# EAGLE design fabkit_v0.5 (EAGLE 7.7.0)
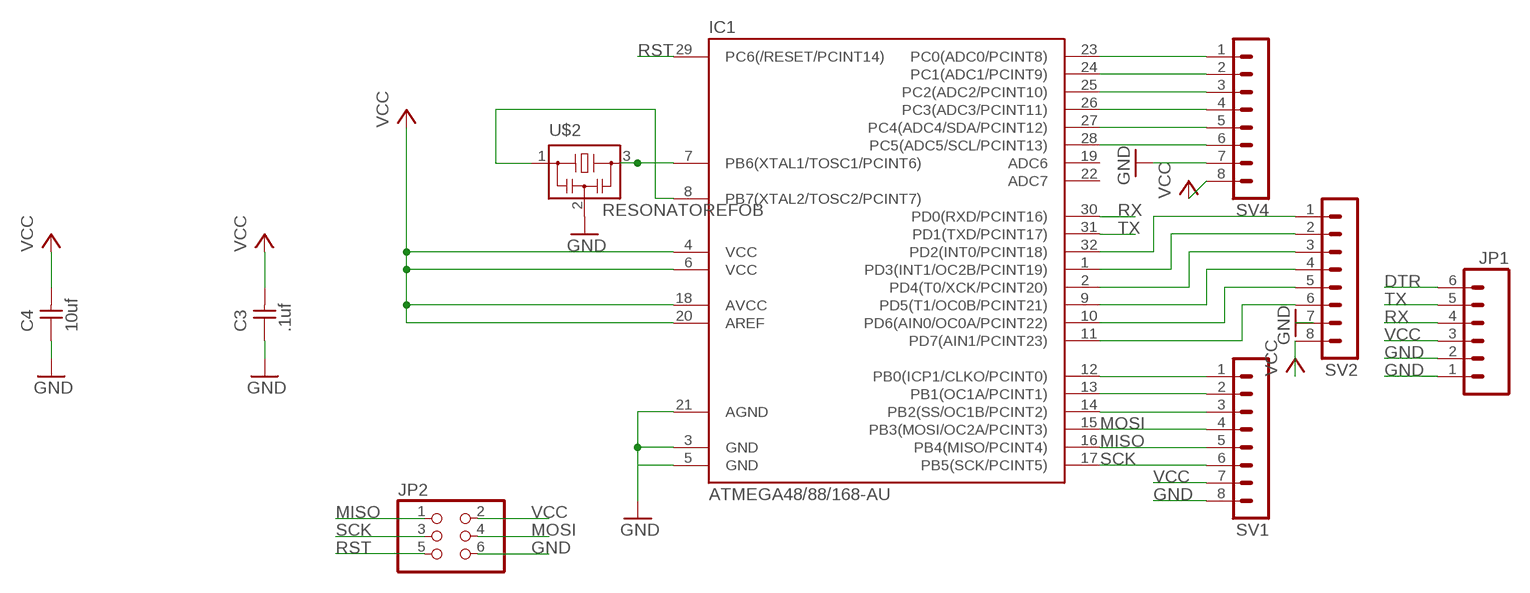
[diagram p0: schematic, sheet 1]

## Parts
C3  .1uf  UNPOLARIZED_CAPACITOR1206  [1206]
C4  10uf  UNPOLARIZED_CAPACITOR1206  [1206]
IC1  ATMEGA48/88/168-AU  [TQFP32-08]
JP1  M06SMD  [1X06-SMD]
JP2  PINHD-2X3-SMD  [2X03SMD]
SV1  MA08-1  [MA08-1]
SV2  MA08-1  [MA08-1]
SV4  MA08-1  [MA08-1]
U$2  RESONATOREFOB  [EFOBM]

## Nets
DTR: JP1.6
GND: C3.1 C4.1 IC1.3(GND) IC1.5(GND) IC1.21(AGND) JP1.1 JP1.2 JP2.6 SV1.8 SV2.7 SV4.7 U$2.2
MISO: IC1.16(PB4(MISO/PCINT4)) JP2.1 SV1.5
MOSI: IC1.15(PB3(MOSI/OC2A/PCINT3)) JP2.4 SV1.4
N$1: IC1.8(PB7(XTAL2/TOSC2/PCINT7)) U$2.1
N$2: IC1.12(PB0(ICP1/CLKO/PCINT0)) SV1.1
N$3: IC1.23(PC0(ADC0/PCINT8)) SV4.1
N$4: IC1.24(PC1(ADC1/PCINT9)) SV4.2
N$5: IC1.25(PC2(ADC2/PCINT10)) SV4.3
N$6: IC1.26(PC3(ADC3/PCINT11)) SV4.4
N$7: IC1.27(PC4(ADC4/SDA/PCINT12)) SV4.5
N$8: IC1.28(PC5(ADC5/SCL/PCINT13)) SV4.6
N$9: IC1.7(PB6(XTAL1/TOSC1/PCINT6)) U$2.3
N$10: IC1.32(PD2(INT0/PCINT18)) SV2.1
N$11: IC1.1(PD3(INT1/OC2B/PCINT19)) SV2.2
N$12: IC1.2(PD4(T0/XCK/PCINT20)) SV2.3
N$13: IC1.9(PD5(T1/OC0B/PCINT21)) SV2.4
N$14: IC1.10(PD6(AIN0/OC0A/PCINT22)) SV2.5
N$15: IC1.11(PD7(AIN1/PCINT23)) SV2.6
N$17: IC1.13(PB1(OC1A/PCINT1)) SV1.2
N$18: IC1.14(PB2(SS/OC1B/PCINT2)) SV1.3
RST: IC1.29(PC6(/RESET/PCINT14)) JP2.5
RX: IC1.30(PD0(RXD/PCINT16)) JP1.4
SCK: IC1.17(PB5(SCK/PCINT5)) JP2.3 SV1.6
TX: IC1.31(PD1(TXD/PCINT17)) JP1.5
VCC: C3.2 C4.2 IC1.4(VCC) IC1.6(VCC) IC1.18(AVCC) IC1.20(AREF) JP1.3 JP2.2 SV1.7 SV2.8 SV4.8
Unconnected: IC1.19(ADC6) IC1.22(ADC7)

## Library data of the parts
C3 C4 = ng:UNPOLARIZED_CAPACITOR: unpolarized_capacitor
IC1 = atmega8:ATMEGA48/88/168
JP1 = SparkFun:M06: Header 6 Standard 6-pin 0.1" header. Use with straight break away headers (SKU : PRT-00116), right angle break away headers (PRT-00553), swiss pins (PRT-00743), machine pins (PRT-00117), and female headers (PRT-00115). Molex polarized connector foot print use with SKU : PRT-08094 with associated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
JP2 = 01_fab:PINHD-2X3-SMD: PIN HEADER
SV1 SV2 SV4 = con-lstb:MA08-1: PIN HEADER
U$2 = fab:RESONATOR

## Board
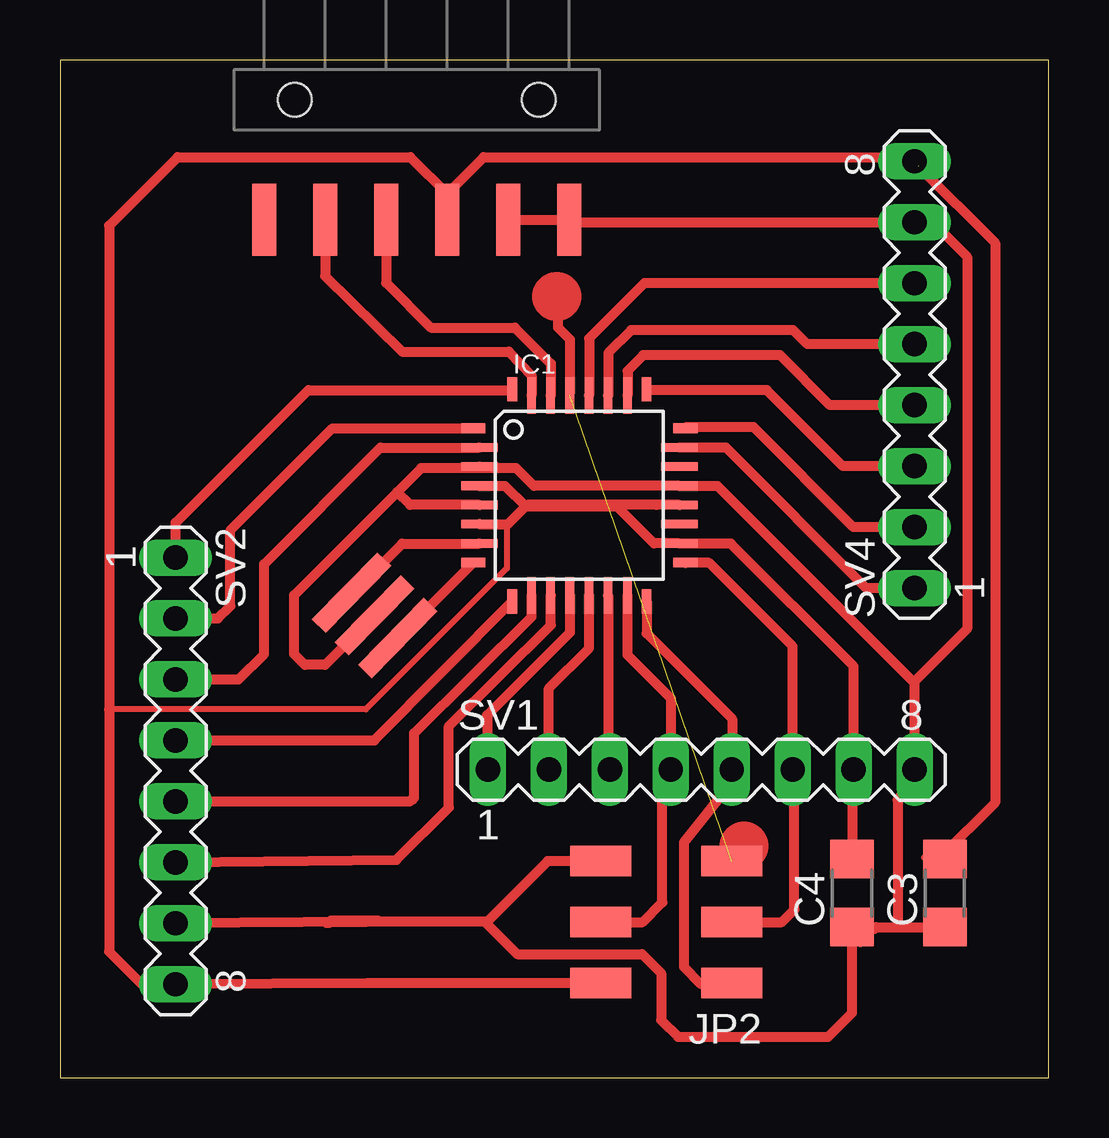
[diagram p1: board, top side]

Size 41.2 x 42.4 mm. Coordinates in mm from the lower left corner, seen from the top.
Outline: 0,0 41.2,0 41.2,42.4 0,42.4 0,0
Copper layers (1*16): Top 0.035mm / dielectric 1.5mm / Bottom 0.035mm
Design rules "default": minimum track width 10mil, minimum drill 24mil, track to track 8mil, track to pad 8mil, pad to pad 8mil, via to via 8mil, smd to smd 8mil, copper to edge 40mil, drill to drill 8mil, minimum pad ring 10mil, minimum via ring 8mil, stop-mask expansion 4mil, vias tented up to drill 0mil, thermal gap 10mil

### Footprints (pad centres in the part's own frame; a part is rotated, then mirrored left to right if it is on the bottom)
1206 = smd 1.6 x 1.803: 1 -1.422,0; 2 1.422,0
TQFP32-08 = smd 1.016 x 0.406: 1 -4.42,2.8; 8 -4.42,-2.8; 17 4.42,-2.8; 24 4.42,2.8 | smd 1.524 x 0.356: 2 -4.166,2; 3 -4.166,1.2; 4 -4.166,0.4; 5 -4.166,-0.4; 6 -4.166,-1.2; 7 -4.166,-2; 18 4.166,-2; 19 4.166,-1.2; 20 4.166,-0.4; 21 4.166,0.4; 22 4.166,1.2; 23 4.166,2 | smd 0.406 x 1.016: 9 -2.8,-4.42; 16 2.8,-4.42; 25 2.8,4.42; 32 -2.8,4.42 | smd 0.356 x 1.524: 10 -2,-4.166; 11 -1.2,-4.166; 12 -0.4,-4.166; 13 0.4,-4.166; 14 1.2,-4.166; 15 2,-4.166; 26 2,4.166; 27 1.2,4.166; 28 0.4,4.166; 29 -0.4,4.166; 30 -1.2,4.166; 31 -2,4.166
1X06-SMD = smd 1 x 3: 1 -6.35,5; 2 -3.81,5; 3 -1.27,5; 4 1.27,5; 5 3.81,5; 6 6.35,5 | hole 1.4: -5.08,0; 5.08,0
2X03SMD = smd 2.54 x 1.27: 1 -2.54,2.54; 2 2.92,2.54; 3 -2.54,0; 4 2.92,0; 5 -2.54,-2.54; 6 2.92,-2.54
MA08-1 = drill 1.016 long: 1 -8.89,0; 2 -6.35,0; 3 -3.81,0; 4 -1.27,0; 5 1.27,0; 6 3.81,0; 7 6.35,0; 8 8.89,0
EFOBM = smd 0.8 x 3.9: 1 -1.35,0; 2 0,0; 3 1.35,0

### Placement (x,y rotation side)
C3  36.87,7.69 90 top
C4  33,7.69 90 top
IC1  21.64,24.26 0 top
JP1  14.86,40.74 180 top
JP2  25.45,6.48 180 top
SV1  26.72,12.83 0 top
SV2  4.82,12.78 270 top
SV4  35.61,29.29 90 top
U$2  13.11,19.26 135.5 top

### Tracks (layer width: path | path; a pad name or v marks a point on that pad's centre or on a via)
GND
  Top 0.254: 33.93,6.2 33.48,5.74 C4.1 | 35.76,6.2 C3.1 | 35.53,13.29 SV1.8
  Top 0.406: 17.53,25.4 19,25.4 19.74,24.66 IC1.21 27.39,24.66 35.6,16.45 | 17.53,25.4 IC1.3 | 35.6,16.45 SV1.8 35.69,12.75 34.9,11.56 34.9,6.27 | JP2.6 20.32,9.02 17.8,6.5 17.7,6.5 | 17.7,6.5 13.3,6.5 | 13.3,6.5 12.8,6.5 | 12.8,6.5 SV2.7 | 11.1,6.45 11.2,6.45 11.3,6.55 | 11.3,6.55 13.25,6.55 13.3,6.5 | U$2.2 13.11,19.16 13.1,19.15 13,19.15 11.05,17.2 10.2,17.2 9.75,17.65 9.75,20.1 14.05,24.4 | IC1.5 14.59,23.86 14.05,24.4 | 17.53,25.4 15.05,25.4 14.05,24.4 | 33.35,5.65 33,6 C4.1 33,2.7 32,1.7 25.75,1.7 25.05,2.4 25.05,4.35 24.25,5.15 19.05,5.15 17.7,6.5 | 11.3,6.55 11.35,6.5 12.8,6.5 | 33.93,6.2 34,6.27 34.9,6.27 | 34.9,6.27 C3.1 | 35.6,16.45 35.6,16.5 37.8,18.7 37.8,34.2 36.4,35.6 35.65,35.6 SV4.7 21.31,35.64 JP1.1 JP1.2
MISO
  Top 0.406: JP2.1 27.95,3.9 26.7,3.9 26,4.6 26,9.8 27.99,12.29 SV1.5 28,14.95 24.44,18.51 IC1.16
MOSI
  Top 0.406: JP2.4 24.28,6.48 25.1,7.3 25.1,12.48 SV1.4 25.45,15.8 23.64,17.61 IC1.15
N$1
  Top 0.406: U$2.1 IC1.8
N$2
  Top 0.406: IC1.12 21.24,18.54 17.8,15.1 17.8,12.86 SV1.1
N$3
  Top 0.406: SV4.1 33.6,20.4 27.75,26.25 IC1.23
N$4
  Top 0.406: SV4.2 33.06,22.94 28.9,27.1 26.1,27.1 IC1.24
N$5
  Top 0.406: SV4.3 32.62,25.48 29.45,28.65 24.47,28.65 IC1.25
N$6
  Top 0.406: SV4.4 32.08,28.02 30,30.1 24.3,30.1 23.65,29.45 IC1.26
N$7
  Top 0.406: SV4.5 31.14,30.56 30.55,31.15 23.8,31.15 22.85,30.2 IC1.27
N$8
  Top 0.406: SV4.6 24.35,33.1 22.05,30.8 IC1.28
N$9
  Top 0.406: U$2.3 12.21,20.21 14.25,22.25 IC1.7
N$10
  Top 0.406: SV2.1 4.82,23.12 10.35,28.65 18.81,28.65 IC1.32
N$11
  Top 0.406: IC1.1 11.35,27.05 7.1,22.8 7.1,19.65 6.58,19.13 SV2.2
N$12
  Top 0.406: SV2.3 7.44,16.59 8.5,17.65 8.5,21.4 13.35,26.25 IC1.2
N$13
  Top 0.406: SV2.4 13.1,14.05 IC1.9
N$14
  Top 0.406: SV2.5 14.56,11.51 14.75,11.65 14.75,14.35 19.65,19.2 IC1.10
N$15
  Top 0.406: SV2.6 14.02,9.07 16.2,11.25 16.2,14.65 20.45,18.85 IC1.11
N$17
  Top 0.406: SV1.2 20.37,16.22 22.05,17.9 IC1.13
N$18
  Top 0.406: IC1.14 22.84,12.9 SV1.3
N$19
  Top 0.406: 21.25,28.55 21.25,30.75 20.75,31.25 20.75,32.5
RST  (1 unrouted)
RX
  Top 0.406: JP1.4 13.59,33.11 15.45,31.25 18.95,31.25 20.45,29.75 IC1.30
SCK
  Top 0.406: JP2.3 30.08,6.48 30.6,7 30.6,12.76 SV1.6 30.53,17.97 27.05,21.45 IC1.17
TX
  Top 0.406: JP1.5 11.05,33.4 14.25,30.25 18.7,30.25 19.65,29.25 IC1.31
VCC  (1 unrouted)
  Top 0.254: 36.68,9.17 35.99,9.17 C3.2 | 35.76,37.98 SV4.8 | 2.05,15.35 12.74,15.35 18.62,21.22 18.62,22.89 18.66,23.06
  Top 0.406: 24.86,23.86 IC1.20 19.46,23.86 19.4,23.8 | IC1.6 18.66,23.06 19.4,23.8 | IC1.4 18.54,24.66 19.4,23.8 | 19.4,23.8 23.2,23.8 24.74,22.26 IC1.18 27.95,22.25 33.07,17.13 SV1.7 | 23.31,3.94 JP2.2 12.82,3.94 SV2.8 3.41,3.89 2.05,5.25 2.05,15.35 2.05,35.5 4.9,38.35 14.6,38.35 16.15,36.8 | 33.05,12.81 SV1.7 | SV1.7 33,12.76 C4.2 33.13,9.11 | 36.68,9.17 38.96,11.46 38.96,34.78 35.76,37.98 | 16.15,36.8 16.15,36.65 16.13,36.63 JP1.3 | 16.15,36.8 16.15,36.85 17.65,38.35 35.4,38.35 35.75,38
(copper drawn outside any net)
  shapes: Top circle x2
